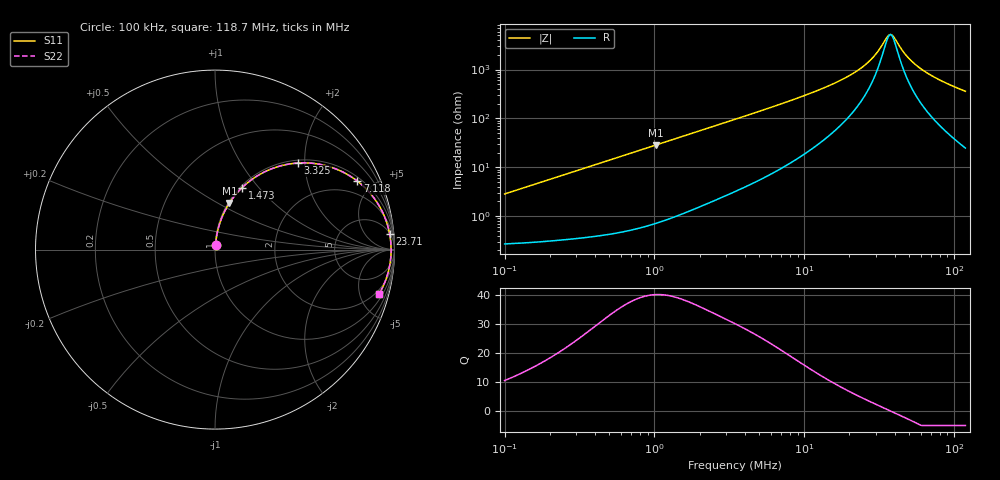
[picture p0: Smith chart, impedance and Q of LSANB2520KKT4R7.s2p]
! LSANB2520KKT4R7  S-PARAMETER MODEL  ( General Type )
! Model Generated by TAIYO YUDEN Corporation (http://www.ty-top.com)
! Version 2.0
! TAIYO YUDEN Control No. 20210629
! Copyright(c) 2013 TAIYO YUDEN CO.,LTD. All Rights Reserved.
! Product Description (link to TY-COMPAS)
! https://ds.yuden.co.jp/TYCOMPAS/or/detail?pn=LSANB2520KKT4R7M&u=M
! Products Name : Inductors
! Characteristics :
!  Inductance : 4.7 uH , SRF(min) : -Hz , DC Resistance(max) : 0.3 Ohm
!  Rated Current : Saturation :1300 mA , Temp Rise : 1100 mA (40 degC)
!  Case Size : 2.5 x 2.0 / 0.098 x 0.079 [mm/inch] , Thickness : 1 / 0.039 [mm/inch]
!  (Conditions: Temperature = 25 degC , DC Bias Current/Voltage = 0A / 0V)
! External Node Assignments :
!  1  o---GGG---o  2
! GND o---------o GND
! Frequency Range : 0.1MHz  -  118.695536MHz  [ 402 STEP ]
# MHz S RI R 50
! Freq[MHz].  S11 Real  S11 Imag  S21 Real  S21 Imag  S12 Real  S12 Imag  S22 Real  S22 Imag
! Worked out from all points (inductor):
!   401 points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, 100 kHz to 118.7 MHz, reference 50 ohm
!   read as one part in series: L = 4.5 uH near 103.6 kHz
!   highest Q = 40.1 at 1.016 MHz (marker M1), where L = 4.44 uH
!   self-resonance near 37.54 MHz
!   S11 on the Smith chart (normalised r, x): 100 kHz: 1.01, +0.06; 1.473 MHz: 1.02, +0.82; 3.325 MHz: 1.06, +1.85; 7.118 MHz: 1.19, +4.04; 23.71 MHz: 5, +21; 118.7 MHz: 1.49, -7.18
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0.1  0.00349 0.0282  0.9965 -0.0282  0.9965 -0.0282  0.00349 0.0282
0.327316  0.0119 0.0905  0.9881 -0.0905  0.9881 -0.0905  0.0119 0.0905
0.58696  0.0305 0.1586  0.9695 -0.1586  0.9695 -0.1586  0.0305 0.1586
1.015962  0.08 0.2591  0.92 -0.2591  0.92 -0.2591  0.08 0.2591
1.07136  0.0878 0.2708  0.9122 -0.2708  0.9122 -0.2708  0.0878 0.2708
1.473279  0.1506 0.345  0.8494 -0.345  0.8494 -0.345  0.1506 0.345
2.174598  0.2735 0.4318  0.7265 -0.4318  0.7265 -0.4318  0.2735 0.4318
3.325409  0.462 0.4824  0.538 -0.4824  0.538 -0.4824  0.462 0.4824
3.445222  0.4792 0.4832  0.5208 -0.4832  0.5208 -0.4832  0.4792 0.4832
4.822284  0.6395 0.4614  0.3605 -0.4614  0.3605 -0.4614  0.6395 0.4614
7.117815  0.7922 0.3823  0.2078 -0.3823  0.2078 -0.3823  0.7922 0.3823
11.27678  0.904 0.2611  0.096 -0.2611  0.096 -0.2611  0.904 0.2611
17.24452  0.9549 0.1567  0.0451 -0.1567  0.0451 -0.1567  0.9549 0.1567
23.71377  0.9729 0.0885  0.0271 -0.0885  0.0271 -0.0885  0.9729 0.0885
29.3247  0.9789 0.0467  0.0211 -0.0467  0.0211 -0.0467  0.9789 0.0467
35.62711  0.9811 0.00982  0.0189 -0.00982  0.0189 -0.00982  0.9811 0.00982
36.91074  0.9812 0.00317  0.0188 -0.00317  0.0188 -0.00317  0.9812 0.00317
38.92342  0.9812 -0.0068  0.0188 0.0068  0.0188 0.0068  0.9812 -0.0068
48.13312  0.9791 -0.047  0.0209 0.047  0.0209 0.047  0.9791 -0.047
59.52193  0.9732 -0.0889  0.0268 0.0889  0.0268 0.0889  0.9732 -0.0889
80.41563  0.9567 -0.1533  0.0433 0.1533  0.0433 0.1533  0.9567 -0.1533
118.6955  0.9135 -0.2487  0.0865 0.2487  0.0865 0.2487  0.9135 -0.2487
